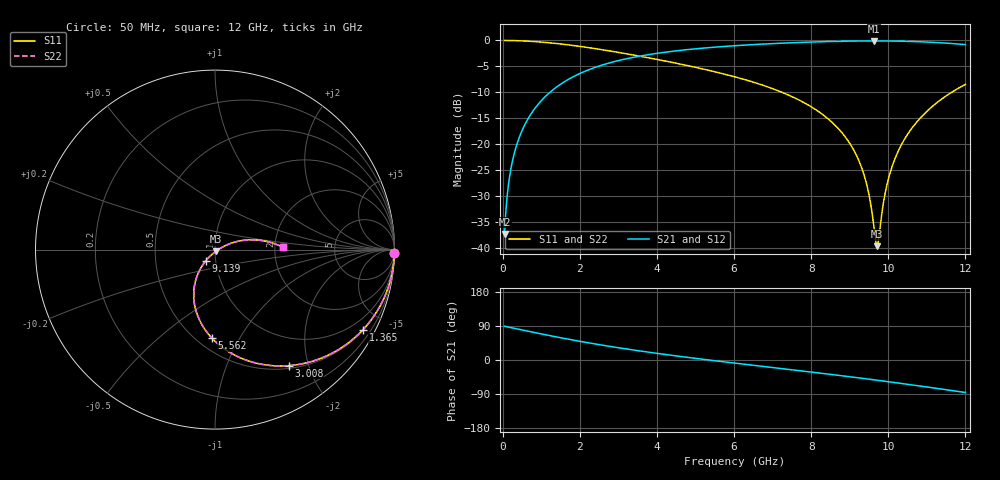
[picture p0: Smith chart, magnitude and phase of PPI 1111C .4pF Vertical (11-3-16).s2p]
# GHz S MA R 50
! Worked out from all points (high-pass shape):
!   1601 points, 50 MHz to 12 GHz, reference 50 ohm
!   highest |S21| = -0.09 dB at 9.632 GHz (marker M1); lowest = -37.4 dB at 50 MHz (marker M2)
!   |S21| within 3 dB of the highest: 3.503 GHz to end of sweep
!   lowest |S11| = -39.7 dB at 9.707 GHz (marker M3), VSWR 1.02, Z = 50.6 - j0.855 ohm
!   |S11| at or under -10 dB: 7.24 GHz to 11.65 GHz (4.405 GHz wide, 46.7 % of centre)
!   |S22| runs from -39.7 to 0.0 dB; largest |S21 - S12| = 0
!   S11 on the Smith chart (normalised r, x): 50 MHz: open; 1.365 GHz: 0.53, -3.87; 3.008 GHz: 0.54, -1.69; 5.562 GHz: 0.59, -0.77; 9.139 GHz: 0.89, -0.11; 12 GHz: 2.21, +0.07
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0.05  0.9999 -1.1  0.01354 88.9  0.01354 88.9  0.9999 -1.1
0.2068437  0.9984 -4.4  0.05593 85.6  0.05593 85.6  0.9984 -4.4
0.4309062  0.9932 -9.2  0.1159 80.8  0.1159 80.8  0.9932 -9.2
0.8118125  0.9765 -17.3  0.215 72.7  0.215 72.7  0.9765 -17.3
1.3645  0.9372 -28.5  0.3477 61.5  0.3477 61.5  0.9372 -28.5
2.044156  0.8721 -41.3  0.4876 48.6  0.4876 48.6  0.8721 -41.3
3.007625  0.7662 -57.6  0.64 32.3  0.64 32.3  0.7662 -57.6
4.038312  0.6522 -72.7  0.7545 17.0  0.7545 17.0  0.6522 -72.7
5.561937  0.4926 -92.1  0.8651 -2.7  0.8651 -2.7  0.4926 -92.1
6.025  0.445 -97.6  0.8899 -8.3  0.8899 -8.3  0.445 -97.6
8.019156  0.2267 -120.0  0.9658 -32.0  0.9658 -32.0  0.2267 -120.0
8.676406  0.1446 -126.6  0.9804 -40.1  0.9804 -40.1  0.1446 -126.6
9.139469  0.08259 -129.4  0.9868 -45.9  0.9868 -45.9  0.08259 -129.4
9.438219  0.04097 -125.8  0.9889 -49.8  0.9889 -49.8  0.04097 -125.8
9.632406  0.01529 -100.5  0.9893 -52.3  0.9893 -52.3  0.01529 -100.5
9.707094  0.01032 -54.9  0.9892 -53.3  0.9892 -53.3  0.01032 -54.9
9.751906  0.01221 -22.2  0.9891 -53.9  0.9891 -53.9  0.01221 -22.2
9.886344  0.02878 12.7  0.9885 -55.7  0.9885 -55.7  0.02878 12.7
10.01331  0.04751 19.4  0.9876 -57.4  0.9876 -57.4  0.04751 19.4
10.29712  0.09154 21.6  0.984 -61.3  0.984 -61.3  0.09154 21.6
10.70791  0.158 18.6  0.975 -67.0  0.975 -67.0  0.158 18.6
12  0.3766 2.1  0.9118 -85.7  0.9118 -85.7  0.3766 2.1
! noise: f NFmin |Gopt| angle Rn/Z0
0.05  0.002035  0.9866  1.051  0.03461
1.372  0.005893  0.7996  12.47  0.006021
2.701  0.009459  0.7482  19.39  0.007352
4.031  0.01279  0.7258  26.28  0.0088
5.36  0.01608  0.7166  33.03  0.01033
6.682  0.01945  0.716  39.52  0.01202
8.012  0.02304  0.7218  45.78  0.014
9.341  0.02699  0.7327  51.73  0.0164
10.67  0.03143  0.7477  57.39  0.0194
12  0.03655  0.7659  62.77  0.02329
